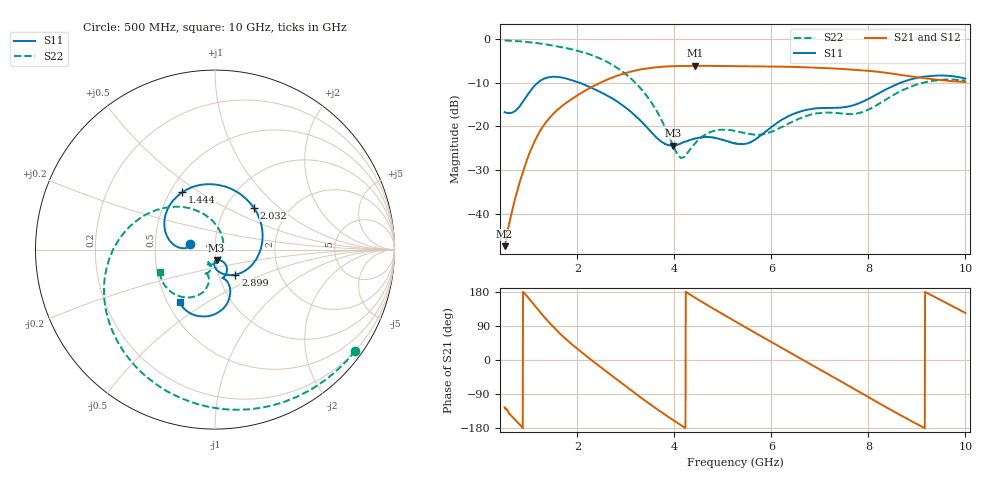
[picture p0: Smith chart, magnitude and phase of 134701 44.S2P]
!  2-Port S-parameters saved by WinCal
! VAR MeasName=S-Parameters (CALIBRATED_DATA) read from VNA (N5242A)
! VAR MeasDate=2013-7-3 16:38:06
! VAR NAME=134701 44
! VAR FILENAME=134701 44.S2P
! VAR DATE=2013-7-3 16:38:06
! VAR PHYS_PORTS=1,2
# Hz S MA R 50
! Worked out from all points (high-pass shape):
!   1601 points, 500 MHz to 10 GHz, reference 50 ohm
!   highest |S21| = -6.13 dB at 4.425 GHz (marker M1); lowest = -47.4 dB at 500 MHz (marker M2)
!   |S21| within 3 dB of the highest: 2.647 GHz to 9.281 GHz (6.634 GHz wide, 111 % of centre)
!   lowest |S11| = -24.4 dB at 3.973 GHz (marker M3), VSWR 1.13, Z = 50.5 - j6.06 ohm
!   |S11| at or under -10 dB: start of sweep to 1.182 GHz; 2.043 GHz to 8.666 GHz (6.623 GHz wide, 124 % of centre)
!   |S22| runs from -27.2 to -0.3 dB; largest |S21 - S12| = 0.002
!   S11 on the Smith chart (normalised r, x): 500 MHz: 0.75, +0.05; 1.444 GHz: 0.58, +0.43; 2.032 GHz: 1.34, +0.70; 2.899 GHz: 1.20, -0.35; 10 GHz: 0.58, -0.39
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5e8  0.1456 167.1  0.004273 -125.0  0.004199 -125.6  0.963 -35.9
9.690625e8  0.2276 173.8  0.04281 167.1  0.0428 167.0  0.9259 -69.1
1.2125e9  0.3262 149.6  0.08525 129.4  0.08516 129.2  0.8913 -86.3
1.444062e9  0.368 119.6  0.1286 95.4  0.1282 95.2  0.8507 -102.1
1.71125e9  0.3593 85.6  0.1759 61.2  0.1755 61.2  0.799 -120.2
2.031875e9  0.3178 47.1  0.2329 26.2  0.2322 26.2  0.7271 -142.3
2.085312e9  0.3101 40.7  0.2427 20.7  0.2421 20.7  0.7138 -146.0
2.459375e9  0.2496 -2.9  0.3136 -16.8  0.3131 -16.7  0.6018 -172.8
2.89875e9  0.18 -50.9  0.3935 -59.9  0.3931 -59.8  0.4376 154.3
3.290625e9  0.1184 -83.3  0.4468 -97.3  0.4474 -97.3  0.2777 123.0
3.670625e9  0.07166 -92.7  0.4785 -132.2  0.478 -132.2  0.1384 87.9
3.973438e9  0.06041 -82.0  0.4892 -158.5  0.4892 -158.6  0.06033 39.9
4.1575e9  0.06502 -76.9  0.4927 -173.9  0.4924 -173.9  0.04381 -16.1
4.424688e9  0.07284 -78.3  0.4937 164.6  0.4936 164.6  0.06363 -74.2
4.780938e9  0.07501 -84.6  0.4925 137.0  0.4924 137.0  0.08766 -105.9
5.25e9  0.06405 -81.4  0.4894 102.0  0.4899 102.0  0.08896 -122.2
6.146562e9  0.1128 -55.6  0.4837 36.8  0.4839 36.8  0.09449 -104.9
6.835312e9  0.1585 -70.4  0.4723 -13.1  0.4725 -13.1  0.1378 -107.9
7.64875e9  0.1726 -71.9  0.4475 -72.3  0.4484 -72.3  0.1386 -112.0
8.420625e9  0.2748 -72.7  0.407 -128.8  0.4067 -128.8  0.2128 -102.2
9.139062e9  0.3706 -94.8  0.3572 -178.4  0.3582 -178.5  0.3168 -123.2
1e10  0.3529 -123.9  0.3228 123.9  0.3231 123.9  0.3329 -157.8
